| Teraspeed Modeling Services.
| http://www.teraspeed.com
[IBIS Ver]  3.2
[File Name] adc12d1600qml.ibs
[File Rev]  3.1
[Source]  Created by Teraspeed Consulting Group LLC
[Date]   05/03/2013
[Notes]   Quality Check of this IBIS model: Model Passes IBIS Check
   Model parses into ICX IS. Simulation done with Hyperlynx.
   1. MIN TYP MAX information is based on Temperature and
   Voltage characteristics only.
   2. Package data gained using TDA Systems IConnect Software.
[Disclaimer]
|[Disclaimer]
|(C) Copyright Texas Instruments Corporation 2013
|   All rights reserved
|   Texas Instruments Corporation hereby grants
|the user of this IBIS model a non-exclusive, nontransferable
|license to use this IBIS model under the following terms.
|Before using this IBIS model, the user should read this
|license.  If the user does not accept these terms,  the
|IBIS model should be returned to Texas Instruments within 30
|days.
|   The user is granted this license only to use the
|IBIS model and is not granted rights to sell, load, rent,
|lease or license the IBIS model in whole or in part, or in
|modified form to anyone other than user. User may modify
|the IBIS model to suit its specific applications but rights
|to derivative works and such modifications shall belong to
|Texas Instruments.
|   This IBIS model is provided on an "AS IS" basis and
|Texas Instruments makes absolutely no warranty with respect to
|the information contained herein.Texas Instruments DISCLAIMS AND
|CUSTOMER WAIVES ALL WARRANTIES, EXPRESS OR IMPLIED, INCLUDING
|WARRANTIES OF MERCHANTABILITY OR FITNESS FOR A PARTICULAR
|PURPOSE. The entire risk as to quality and performance is
|with the Customer. ACCORDINGLY, IN NO EVENT SHALL THE
|COMPANY BE LIABLE FOR ANY DAMAGES, WHETHER IN CONTRACT OR
|TORT,INCLUDING ANY LOST PROFITS OR OTHER INCIDENTAL,
|CONSEQUENTIAL, EXEMPLARY, OR PUNITIVE DAMAGES ARISING OUT
|OF THE USE OR APPLICATION OF THE IBIS model provided in
|this package.Further, Texas Instruments reserves the right to
|make changes without notice to any product herein to improve
|reliability, function, or design. Texas Instruments does not
|convey any license under patent rights or any other intellectual
|property rights, including those of third parties.
|   Texas Instruments is not obligated to provide maintenance
|or support for the licensed IBIS model.
| Use: Teraspeed Consulting Group LLC ("Teraspeed") has
| licensed IBIS models to specific integrated circuit
| suppliers ("IC Vendors") for use and distribution as
| follows: Each IC Vendor may use IBIS Models, and distribute
| them to IC Vendor's custumers to use solely for developing
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[Copyright]
| This file is the legal property of Texas Instruments and
| Teraspeed Copyright(c) 2013.
| All other rights are reserved.
[Component]   ADC12D1600QML
[Manufacturer] Texas Instruments
[Package]
| variable   typ   min   max
R_pkg  7.571E-03  2.653E-03   1.171E-02
L_pkg  3.048E-09  8.840E-10   1.031E-08
C_pkg  1.181E-12  2.940E-13   4.159E-12
[Pin] signal_name  model_name  R_pin  L_pin C_pin
A1   GND   GND   1.171E-02 8.840E-10 2.940E-13
A2   V_A   POWER   1.083E-02 8.840E-10 2.940E-13
A3   SDO   out_tri   1.000E-02 8.934E-09 3.594E-12
A4   TPM   input   9.232E-03 8.316E-09 3.340E-12
A5   NDM   input   8.534E-03 7.754E-09 3.110E-12
A6   V_A   POWER   7.917E-03 8.840E-10 2.940E-13
A7   GND   GND   7.392E-03 8.840E-10 2.940E-13
A8   V_E   POWER   6.969E-03 8.840E-10 2.940E-13
A9   GND_E   GND   6.659E-03 8.840E-10 2.940E-13
A10   DId0+   lvds_hs   6.469E-03 6.092E-09 2.429E-12
A11   V_DR   POWER   6.469E-03 8.840E-10 2.940E-13
A12   DId3+   lvds_hs   6.659E-03 6.244E-09 2.491E-12
A13   GND_DR   GND   6.969E-03 8.840E-10 2.940E-13
A14   DId6+   lvds_hs   7.392E-03 6.835E-09 2.733E-12
A15   V_DR   POWER   7.917E-03 8.840E-10 2.940E-13
A16   DId9+   lvds_hs   8.534E-03 7.754E-09 3.110E-12
A17   GND_DR   GND   9.232E-03 8.840E-10 2.940E-13
A18   DId11+   lvds_hs   1.000E-02 8.934E-09 3.594E-12
A19   DId11-   lvds_hs   1.083E-02 9.602E-09 3.868E-12
A20   GND_DR   GND   1.171E-02 8.840E-10 2.940E-13
B1   Vbg   term   1.083E-02 9.602E-09 3.868E-12
B2   GND   GND   9.900E-03 8.840E-10 2.940E-13
B3   ECEb   in_pu   9.020E-03 8.145E-09 3.271E-12
B4   SDI   input   8.201E-03 7.486E-09 3.000E-12
B5   CalRun   output   7.451E-03 6.882E-09 2.753E-12
B6   V_A   POWER   6.784E-03 8.840E-10 2.940E-13
B7   GND   GND   6.212E-03 8.840E-10 2.940E-13
B8   GND_E   GND   5.748E-03 8.840E-10 2.940E-13
B9   V_E   POWER   5.405E-03 8.840E-10 2.940E-13
B10   DId0-   lvds_hs   5.195E-03 5.066E-09 2.008E-12
B11   DId2+   lvds_hs   5.195E-03 5.066E-09 2.008E-12
B12   DId3-   lvds_hs   5.405E-03 5.235E-09 2.078E-12
B13   DId5+   lvds_hs   5.748E-03 5.511E-09 2.191E-12
B14   DId6-   lvds_hs   6.212E-03 5.884E-09 2.344E-12
B15   DId8+   lvds_hs   6.784E-03 6.345E-09 2.533E-12
B16   DId9-   lvds_hs   7.451E-03 6.882E-09 2.753E-12
B17   DId10+   lvds_hs   8.201E-03 7.486E-09 3.000E-12
B18   DI0+   lvds_hs   9.020E-03 8.145E-09 3.271E-12
B19   DI1+   lvds_hs   9.900E-03 8.853E-09 3.561E-12
B20   DI1-   lvds_hs   1.083E-02 9.602E-09 3.868E-12
C1   Rtrim+   term   1.000E-02 8.934E-09 3.594E-12
C2   GND   GND   9.020E-03 8.145E-09 3.271E-12
C3   Rext+   term   8.088E-03 7.395E-09 2.963E-12
C4   SCSb   input   7.212E-03 6.690E-09 2.674E-12
C5   SCLK   input   6.405E-03 6.040E-09 2.408E-12
C6   GND   GND   5.680E-03 8.840E-10 2.940E-13
C7   V_A   POWER   5.053E-03 8.840E-10 2.940E-13
C8   V_E   POWER   4.540E-03 8.840E-10 2.940E-13
C9   GND_E   GND   4.158E-03 8.840E-10 2.940E-13
C10   DId1+   lvds_hs   3.923E-03 4.042E-09 1.589E-12
C11   DId2-   lvds_hs   3.923E-03 4.042E-09 1.589E-12
C12   DId4+   lvds_hs   4.158E-03 4.232E-09 1.666E-12
C13   DId5-   lvds_hs   4.540E-03 4.539E-09 1.792E-12
C14   DId7+   lvds_hs   5.053E-03 4.951E-09 1.961E-12
C15   DId8-   lvds_hs   5.680E-03 5.456E-09 2.168E-12
C16   DId10-   lvds_hs   6.405E-03 6.040E-09 2.408E-12
C17   DI0-   lvds_hs   7.212E-03 6.690E-09 2.674E-12
C18   V_DR   POWER   8.088E-03 8.840E-10 2.940E-13
C19   DI12+   lvds_hs   9.020E-03 8.145E-09 3.271E-12
C20   DI12-   lvds_hs   1.000E-02 8.934E-09 3.594E-12
D1   V_A   POWER   9.232E-03 8.316E-09 3.340E-12
D2   Rtrim-   term   8.201E-03 7.486E-09 3.000E-12
D3   Rext-   term   7.212E-03 6.690E-09 2.674E-12
D4   GND   GND   6.276E-03 8.840E-10 2.940E-13
D5   GND   GND   5.405E-03 8.840E-10 2.940E-13
D6   CAL   input   4.615E-03 4.599E-09 1.817E-12
D7   Vbiasl   term   3.923E-03 4.042E-09 1.589E-12
D8   V_A   POWER   3.351E-03 8.840E-10 2.940E-13
D9   V_A   POWER   2.921E-03 8.840E-10 2.940E-13
D10   DId1-   lvds_hs   2.653E-03 3.020E-09 1.170E-12
D11   V_DR   POWER   2.653E-03 8.840E-10 2.940E-13
D12   DId4-   lvds_hs   2.921E-03 3.235E-09 1.258E-12
D13   GND_DR   GND   3.351E-03 8.840E-10 2.940E-13
D14   DId7-   lvds_hs   3.923E-03 4.042E-09 1.589E-12
D15   V_DR   POWER   4.615E-03 8.840E-10 2.940E-13
D16   GND_DR   GND   5.405E-03 8.840E-10 2.940E-13
D17   V_DR   POWER   6.276E-03 8.840E-10 2.940E-13
D18   DI3+   lvds_hs   7.212E-03 6.690E-09 2.674E-12
D19   DI4+   lvds_hs   8.201E-03 7.486E-09 3.000E-12
D20   DI4-   lvds_hs   9.232E-03 8.316E-09 3.340E-12
E1   V_A   POWER   8.534E-03 8.840E-10 2.940E-13
E2   Tdiode+   term   7.451E-03 6.882E-09 2.753E-12
E3   RSV1   NC   6.405E-03 6.040E-09 2.408E-12
E4   GND   GND   5.405E-03 8.840E-10 2.940E-13
E17   GND_DR   GND   5.405E-03 8.840E-10 2.940E-13
E18   DI3-   lvds_hs   6.405E-03 6.040E-09 2.408E-12
E19   DI5+   lvds_hs   7.451E-03 6.882E-09 2.753E-12
E20   DI5-   lvds_hs   8.534E-03 7.754E-09 3.110E-12
F1   V_A   POWER   7.917E-03 8.840E-10 2.940E-13
F2   GND_TC   GND   6.784E-03 8.840E-10 2.940E-13
F3   Tdiode-   term   5.680E-03 5.456E-09 2.168E-12
F4   RSV2   NC   4.615E-03 4.599E-09 1.817E-12
F17   GND_DR   GND   4.615E-03 8.840E-10 2.940E-13
F18   DI6+   lvds_hs   5.680E-03 5.456E-09 2.168E-12
F19   DI6-   lvds_hs   6.784E-03 6.345E-09 2.533E-12
F20   GND_DR   GND   7.917E-03 8.840E-10 2.940E-13
G1   V_TC   POWER   7.392E-03 8.840E-10 2.940E-13
G2   GND_TC   GND   6.212E-03 8.840E-10 2.940E-13
G3   V_TC   POWER   5.053E-03 8.840E-10 2.940E-13
G4   V_TC   POWER   3.923E-03 8.840E-10 2.940E-13
G17   DI7+   lvds_hs   3.923E-03 8.840E-10 2.940E-13
G18   DI7-   lvds_hs   5.053E-03 8.951E-10 2.961E-13
G19   DI8+   lvds_hs   6.212E-03 5.884E-09 2.344E-12
G20   DI8-   lvds_hs   7.392E-03 6.835E-09 2.733E-12
H1   Vinl+   term   6.969E-03 6.494E-09 2.594E-12
H2   V_TC   POWER   5.748E-03 8.840E-10 2.940E-13
H3   GND_TC   GND   4.540E-03 8.840E-10 2.940E-13
H4   V_A   POWER   3.351E-03 8.840E-10 2.940E-13
H17   DI9+   lvds_hs   3.351E-03 3.581E-09 1.400E-12
H18   DI9-   lvds_hs   4.540E-03 4.539E-09 1.792E-12
H19   DI10+   lvds_hs   5.748E-03 5.511E-09 2.191E-12
H20   DI10-   lvds_hs   6.969E-03 6.494E-09 2.594E-12
J1   Vinl-   term   6.659E-03 6.244E-09 2.491E-12
J2   GND_TC   GND   5.405E-03 8.840E-10 2.940E-13
J3   V_TC   POWER   4.158E-03 8.840E-10 2.940E-13
J4   VbiasI   term   2.921E-03 3.235E-09 1.258E-12
J17   V_DR   POWER   2.921E-03 8.840E-10 2.940E-13
J18   DI11+   lvds_hs   4.158E-03 4.232E-09 1.666E-12
J19   DI11-   lvds_hs   5.405E-03 5.235E-09 2.078E-12
J20   V_DR   POWER   6.659E-03 8.840E-10 2.940E-13
K1   GND   GND   6.469E-03 8.840E-10 2.940E-13
K2   VbiasI   term   5.195E-03 5.066E-09 2.008E-12
K3   V_TC   POWER   3.923E-03 8.840E-10 2.940E-13
K4   GND_TC   GND   2.653E-03 8.840E-10 2.940E-13
K17   ORI+   lvds_hs   2.653E-03 3.020E-09 1.170E-12
K18   ORI-   lvds_hs   3.923E-03 4.042E-09 1.589E-12
K19   DCLKI+   lvds_hs   5.195E-03 5.066E-09 2.008E-12
K20   DCLKI-   lvds_hs   6.469E-03 6.092E-09 2.429E-12
L1   GND   GND   6.469E-03 8.840E-10 2.940E-13
L2   VbiasQ   term   5.195E-03 5.066E-09 2.008E-12
L3   V_TC   POWER   3.923E-03 8.840E-10 2.940E-13
L4   GND_TC   GND   2.653E-03 8.840E-10 2.940E-13
L17   ORQ+   lvds_hs   2.653E-03 3.020E-09 1.170E-12
L18   ORQ-   lvds_hs   3.923E-03 4.042E-09 1.589E-12
L19   DCLKQ+   lvds_hs   5.195E-03 5.066E-09 2.008E-12
L20   DCLKQ-   lvds_hs   6.469E-03 6.092E-09 2.429E-12
M1   VinQ-   term   6.659E-03 6.244E-09 2.491E-12
M2   GND_TC   GND   5.405E-03 8.840E-10 2.940E-13
M3   V_TC   POWER   4.158E-03 8.840E-10 2.940E-13
M4   VbiasQ   term   2.921E-03 3.235E-09 1.258E-12
M17   GND_DR   GND   2.921E-03 8.840E-10 2.940E-13
M18   DQ11+   lvds_hs   4.158E-03 4.232E-09 1.666E-12
M19   DQ11-   lvds_hs   5.405E-03 5.235E-09 2.078E-12
M20   GND_DR   GND   6.659E-03 8.840E-10 2.940E-13
N1   VinQ+   term   6.969E-03 6.494E-09 2.594E-12
N2   V_TC   POWER   5.748E-03 8.840E-10 2.940E-13
N3   GND_TC   GND   4.540E-03 8.840E-10 2.940E-13
N4   V_A   POWER   3.351E-03 8.840E-10 2.940E-13
N17   DQ9+   lvds_hs   3.351E-03 3.581E-09 1.400E-12
N18   DQ9-   lvds_hs   4.540E-03 4.539E-09 1.792E-12
N19   DQ10+   lvds_hs   5.748E-03 5.511E-09 2.191E-12
N20   DQ10-   lvds_hs   6.969E-03 6.494E-09 2.594E-12
P1   V_TC   POWER   7.392E-03 8.840E-10 2.940E-13
P2   GND_TC   GND   6.212E-03 8.840E-10 2.940E-13
P3   V_TC   POWER   5.053E-03 8.840E-10 2.940E-13
P4   V_TC   POWER   3.923E-03 8.840E-10 2.940E-13
P17   DQ7+   lvds_hs   3.923E-03 4.042E-09 1.589E-12
P18   DQ7-   lvds_hs   5.053E-03 4.951E-09 1.961E-12
P19   DQ8+   lvds_hs   6.212E-03 5.884E-09 2.344E-12
P20   DQ8-   lvds_hs   7.392E-03 6.835E-09 2.733E-12
R1   V_A   POWER   7.917E-03 8.840E-10 2.940E-13
R2   GND_TC   GND   6.784E-03 8.840E-10 2.940E-13
R3   V_TC   POWER   5.680E-03 8.840E-10 2.940E-13
R4   V_TC   POWER   4.615E-03 8.840E-10 2.940E-13
R17   V_DR   POWER   4.615E-03 8.840E-10 2.940E-13
R18   DQ6+   lvds_hs   5.680E-03 5.456E-09 2.168E-12
R19   DQ6-   lvds_hs   6.784E-03 6.345E-09 2.533E-12
R20   V_DR   POWER   7.917E-03 8.840E-10 2.940E-13
T1   V_A   POWER   8.534E-03 8.840E-10 2.940E-13
T2   GND_TC   GND   7.451E-03 8.840E-10 2.940E-13
T3   GND_TC   GND   6.405E-03 8.840E-10 2.940E-13
T4   GND   GND   5.405E-03 8.840E-10 2.940E-13
T17   V_DR   POWER   5.405E-03 8.840E-10 2.940E-13
T18   DQ3-   lvds_hs   6.405E-03 6.040E-09 2.408E-12
T19   DQ5+   lvds_hs   7.451E-03 6.882E-09 2.753E-12
T20   DQ5-   lvds_hs   8.534E-03 7.754E-09 3.110E-12
U1   GND_TC   GND   9.232E-03 8.840E-10 2.940E-13
U2   CLK+   in_clk   8.201E-03 7.486E-09 3.000E-12
U3   PDI   in_pu   7.212E-03 6.690E-09 2.674E-12
U4   GND   GND   6.276E-03 8.840E-10 2.940E-13
U5   GND   GND   5.405E-03 8.840E-10 2.940E-13
U6   RCOut1-   lvds_ls   4.615E-03 4.599E-09 1.817E-12
U7   VbiasQ   term   3.923E-03 4.042E-09 1.589E-12
U8   V_A   POWER   3.351E-03 8.840E-10 2.940E-13
U9   V_A   POWER   2.921E-03 8.840E-10 2.940E-13
U10   DQd1-   lvds_hs   2.653E-03 3.020E-09 1.170E-12
U11   V_DR   POWER   2.653E-03 8.840E-10 2.940E-13
U12   DQd4-   lvds_hs   2.921E-03 3.235E-09 1.258E-12
U13   GND_DR   GND   3.351E-03 8.840E-10 2.940E-13
U14   DQd7-   lvds_hs   3.923E-03 4.042E-09 1.589E-12
U15   V_DR   POWER   4.615E-03 8.840E-10 2.940E-13
U16   V_DR   POWER   5.405E-03 8.840E-10 2.940E-13
U17   GND_DR   GND   6.276E-03 8.840E-10 2.940E-13
U18   DQ3+   lvds_hs   7.212E-03 6.690E-09 2.674E-12
U19   DQ4+   lvds_hs   8.201E-03 7.486E-09 3.000E-12
U20   DQ4-   lvds_hs   9.232E-03 8.316E-09 3.340E-12
V1   CLK-   in_clk   1.000E-02 8.934E-09 3.594E-12
V2   DCLK_RST+ in_clk   9.020E-03 8.145E-09 3.271E-12
V3   PDQ   in_pu   8.088E-03 7.395E-09 2.963E-12
V4   LSPSM   input   7.212E-03 6.690E-09 2.674E-12
V5   DES   input   6.405E-03 6.040E-09 2.408E-12
V6   RCOut2+   lvds_ls   5.680E-03 5.456E-09 2.168E-12
V7   RCOut2-   lvds_ls   5.053E-03 4.951E-09 1.961E-12
V8   V_E   POWER   4.540E-03 8.840E-10 2.940E-13
V9   GND_E   GND   4.158E-03 8.840E-10 2.940E-13
V10   DQd1+   lvds_hs   3.923E-03 4.042E-09 1.589E-12
V11   DQd02-   lvds_hs   3.923E-03 4.042E-09 1.589E-12
V12   DQd4+   lvds_hs   4.158E-03 4.232E-09 1.666E-12
V13   DQd5-   lvds_hs   4.540E-03 4.539E-09 1.792E-12
V14   DQd7+   lvds_hs   5.053E-03 4.951E-09 1.961E-12
V15   DQd8-   lvds_hs   5.680E-03 5.456E-09 2.168E-12
V16   DQd10-   lvds_hs   6.405E-03 6.040E-09 2.408E-12
V17   DQ0-   lvds_hs   7.212E-03 6.690E-09 2.674E-12
V18   GND_DR   GND   8.088E-03 8.840E-10 2.940E-13
V19   DQ2+   lvds_hs   9.020E-03 8.145E-09 3.271E-12
V20   DQ2-   lvds_hs   1.000E-02 8.934E-09 3.594E-12
W1   DCLK_RST- in_clk   1.083E-02 9.602E-09 3.868E-12
W2   GND   GND   9.900E-03 8.840E-10 2.940E-13
W3   RSV   NC   9.020E-03 8.145E-09 3.271E-12
W4   DDRPh   input   8.201E-03 7.486E-09 3.000E-12
W5   RCLK-   in_clk   7.451E-03 6.882E-09 2.753E-12
W6   V_A   POWER   6.784E-03 8.840E-10 2.940E-13
W7   GND   GND   6.212E-03 8.840E-10 2.940E-13
W8   GND_E   GND   5.748E-03 8.840E-10 2.940E-13
W9   V_E   POWER   5.405E-03 8.840E-10 2.940E-13
W10   DQd0-   lvds_hs   5.195E-03 5.066E-09 2.008E-12
W11   DQd2+   lvds_hs   5.195E-03 5.066E-09 2.008E-12
W12   DQd3-   lvds_hs   5.405E-03 5.235E-09 2.078E-12
W13   DQd5+   lvds_hs   5.748E-03 5.511E-09 2.191E-12
W14   DQd6-   lvds_hs   6.212E-03 5.884E-09 2.344E-12
W15   DQd8+   lvds_hs   6.784E-03 6.345E-09 2.533E-12
W16   DQd9-   lvds_hs   7.451E-03 6.882E-09 2.753E-12
W17   DQd10+   lvds_hs   8.201E-03 7.486E-09 3.000E-12
W18   DQ0+   lvds_hs   9.020E-03 8.145E-09 3.271E-12
W19   DQ1+   lvds_hs   9.900E-03 8.853E-09 3.561E-12
W20   DQ1-   lvds_hs   1.083E-02 9.602E-09 3.868E-12
Y1   GND   GND   1.171E-02 8.840E-10 2.940E-13
Y2   V_A   POWER   1.083E-02 8.840E-10 2.940E-13
Y3   FSR   input   1.000E-02 8.934E-09 3.594E-12
Y4   RCLK+   in_clk   9.232E-03 8.316E-09 3.340E-12
Y5   RCOut1+   lvds_ls   8.534E-03 7.754E-09 3.110E-12
Y6   V_A   POWER   7.917E-03 8.840E-10 2.940E-13
Y7   GND   GND   7.392E-03 8.840E-10 2.940E-13
Y8   V_E   POWER   6.969E-03 8.840E-10 2.940E-13
Y9   GND_E   GND   6.659E-03 8.840E-10 2.940E-13
Y10   DQd0+   lvds_hs   6.469E-03 6.092E-09 2.429E-12
Y11   V_DR   POWER   6.469E-03 8.840E-10 2.940E-13
Y12   DQd3+   lvds_hs   6.659E-03 6.244E-09 2.491E-12
Y13   GND_DR   GND   6.969E-03 8.840E-10 2.940E-13
Y14   DQd6+   lvds_hs   7.392E-03 6.835E-09 2.733E-12
Y15   V_DR   POWER   7.917E-03 8.840E-10 2.940E-13
Y16   DQd9+   lvds_hs   8.534E-03 7.754E-09 3.110E-12
Y17   GND_DR   GND   9.232E-03 8.840E-10 2.940E-13
Y18   DQd11+   lvds_hs   1.000E-02 8.934E-09 3.594E-12
Y19   DQd11-   lvds_hs   1.083E-02 9.602E-09 3.868E-12
Y20   GND_DR   GND   1.171E-02 1.031E-08 4.159E-12
AA2   GND   GND   1.000E-02 8.840E-10 2.940E-13
AA3   GND   GND   1.000E-02 8.840E-10 2.940E-13
AA4   GND   GND   1.000E-02 8.840E-10 2.940E-13
AA5   GND   GND   1.000E-02 8.840E-10 2.940E-13
AA6   GND   GND   1.000E-02 8.840E-10 2.940E-13
AA7   GND   GND   1.000E-02 8.840E-10 2.940E-13
AA8   GND   GND   1.000E-02 8.840E-10 2.940E-13
AA9   GND   GND   1.000E-02 8.840E-10 2.940E-13
AA10  GND   GND   1.000E-02 8.840E-10 2.940E-13
AA11  GND   GND   1.000E-02 8.840E-10 2.940E-13
AB1   GND   GND   1.000E-02 8.840E-10 2.940E-13
AB2   GND   GND   1.000E-02 8.840E-10 2.940E-13
AB3   GND   GND   1.000E-02 8.840E-10 2.940E-13
AB4   GND   GND   1.000E-02 8.840E-10 2.940E-13
AB5   GND   GND   1.000E-02 8.840E-10 2.940E-13
AB6   GND   GND   1.000E-02 8.840E-10 2.940E-13
AB7   GND   GND   1.000E-02 8.840E-10 2.940E-13
AB8   GND   GND   1.000E-02 8.840E-10 2.940E-13
AB9   GND   GND   1.000E-02 8.840E-10 2.940E-13
AB10  GND   GND   1.000E-02 8.840E-10 2.940E-13
AB11  GND   GND   1.000E-02 8.840E-10 2.940E-13
AC1   GND   GND   1.000E-02 8.840E-10 2.940E-13
AC2   GND   GND   1.000E-02 8.840E-10 2.940E-13
AC3   GND   GND   1.000E-02 8.840E-10 2.940E-13
AC4   GND   GND   1.000E-02 8.840E-10 2.940E-13
AC5   GND   GND   1.000E-02 8.840E-10 2.940E-13
AC6   GND   GND   1.000E-02 8.840E-10 2.940E-13
AC7   GND   GND   1.000E-02 8.840E-10 2.940E-13
AC8   GND   GND   1.000E-02 8.840E-10 2.940E-13
AC9   GND   GND   1.000E-02 8.840E-10 2.940E-13
AC10  GND   GND   1.000E-02 8.840E-10 2.940E-13
AC11  GND   GND   1.000E-02 8.840E-10 2.940E-13
AD1   GND   GND   1.000E-02 8.840E-10 2.940E-13
AD2   GND   GND   1.000E-02 8.840E-10 2.940E-13
AD3   GND   GND   1.000E-02 8.840E-10 2.940E-13
AD4   GND   GND   1.000E-02 8.840E-10 2.940E-13
AD5   GND   GND   1.000E-02 8.840E-10 2.940E-13
AD6   GND   GND   1.000E-02 8.840E-10 2.940E-13
AD7   GND   GND   1.000E-02 8.840E-10 2.940E-13
AD8   GND   GND   1.000E-02 8.840E-10 2.940E-13
AD9   GND   GND   1.000E-02 8.840E-10 2.940E-13
AD10  GND   GND   1.000E-02 8.840E-10 2.940E-13
AD11  GND   GND   1.000E-02 8.840E-10 2.940E-13
AE1   GND   GND   1.000E-02 8.840E-10 2.940E-13
AE2   GND   GND   1.000E-02 8.840E-10 2.940E-13
AE3   GND   GND   1.000E-02 8.840E-10 2.940E-13
AE4   GND   GND   1.000E-02 8.840E-10 2.940E-13
AE5   GND   GND   1.000E-02 8.840E-10 2.940E-13
AE6   GND   GND   1.000E-02 8.840E-10 2.940E-13
AE7   GND   GND   1.000E-02 8.840E-10 2.940E-13
AE8   GND   GND   1.000E-02 8.840E-10 2.940E-13
AE9   GND   GND   1.000E-02 8.840E-10 2.940E-13
AE10  GND   GND   1.000E-02 8.840E-10 2.940E-13
AE11  GND   GND   1.000E-02 8.840E-10 2.940E-13
AF1   GND   GND   1.000E-02 8.840E-10 2.940E-13
AF2   GND   GND   1.000E-02 8.840E-10 2.940E-13
AF3   GND   GND   1.000E-02 8.840E-10 2.940E-13
AF4   GND   GND   1.000E-02 8.840E-10 2.940E-13
AF5   GND   GND   1.000E-02 8.840E-10 2.940E-13
AF6   GND   GND   1.000E-02 8.840E-10 2.940E-13
AF7   GND   GND   1.000E-02 8.840E-10 2.940E-13
AF8   GND   GND   1.000E-02 8.840E-10 2.940E-13
AF9   GND   GND   1.000E-02 8.840E-10 2.940E-13
AF10  GND   GND   1.000E-02 8.840E-10 2.940E-13
AF11  GND   GND   1.000E-02 8.840E-10 2.940E-13
AG1   GND   GND   1.000E-02 8.840E-10 2.940E-13
AG2   GND   GND   1.000E-02 8.840E-10 2.940E-13
AG3   GND   GND   1.000E-02 8.840E-10 2.940E-13
AG4   GND   GND   1.000E-02 8.840E-10 2.940E-13
AG5   GND   GND   1.000E-02 8.840E-10 2.940E-13
AG6   GND   GND   1.000E-02 8.840E-10 2.940E-13
AG7   GND   GND   1.000E-02 8.840E-10 2.940E-13
AG8   GND   GND   1.000E-02 8.840E-10 2.940E-13
AG9   GND   GND   1.000E-02 8.840E-10 2.940E-13
AG10  GND   GND   1.000E-02 8.840E-10 2.940E-13
AG11  GND   GND   1.000E-02 8.840E-10 2.940E-13
AH1   GND   GND   1.000E-02 8.840E-10 2.940E-13
AH2   GND   GND   1.000E-02 8.840E-10 2.940E-13
AH3   GND   GND   1.000E-02 8.840E-10 2.940E-13
AH4   GND   GND   1.000E-02 8.840E-10 2.940E-13
AH5   GND   GND   1.000E-02 8.840E-10 2.940E-13
AH6   GND   GND   1.000E-02 8.840E-10 2.940E-13
AH7   GND   GND   1.000E-02 8.840E-10 2.940E-13
AH8   GND   GND   1.000E-02 8.840E-10 2.940E-13
AH9   GND   GND   1.000E-02 8.840E-10 2.940E-13
AH10  GND   GND   1.000E-02 8.840E-10 2.940E-13
AH11  GND   GND   1.000E-02 8.840E-10 2.940E-13
AJ1   GND   GND   1.000E-02 8.840E-10 2.940E-13
AJ2   GND   GND   1.000E-02 8.840E-10 2.940E-13
AJ3   GND   GND   1.000E-02 8.840E-10 2.940E-13
AJ4   GND   GND   1.000E-02 8.840E-10 2.940E-13
AJ5   GND   GND   1.000E-02 8.840E-10 2.940E-13
AJ6   GND   GND   1.000E-02 8.840E-10 2.940E-13
AJ7   GND   GND   1.000E-02 8.840E-10 2.940E-13
AJ8   GND   GND   1.000E-02 8.840E-10 2.940E-13
AJ9   GND   GND   1.000E-02 8.840E-10 2.940E-13
AJ10  GND   GND   1.000E-02 8.840E-10 2.940E-13
AJ11  GND   GND   1.000E-02 8.840E-10 2.940E-13
AK1   GND   GND   1.000E-02 8.840E-10 2.940E-13
AK2   GND   GND   1.000E-02 8.840E-10 2.940E-13
AK3   GND   GND   1.000E-02 8.840E-10 2.940E-13
AK4   GND   GND   1.000E-02 8.840E-10 2.940E-13
AK5   GND   GND   1.000E-02 8.840E-10 2.940E-13
AK6   GND   GND   1.000E-02 8.840E-10 2.940E-13
AK7   GND   GND   1.000E-02 8.840E-10 2.940E-13
AK8   GND   GND   1.000E-02 8.840E-10 2.940E-13
AK9   GND   GND   1.000E-02 8.840E-10 2.940E-13
AK10  GND   GND   1.000E-02 8.840E-10 2.940E-13
AK11  GND   GND   1.000E-02 8.840E-10 2.940E-13
AL1   GND   GND   1.000E-02 8.840E-10 2.940E-13
AL2   GND   GND   1.000E-02 8.840E-10 2.940E-13
AL3   GND   GND   1.000E-02 8.840E-10 2.940E-13
AL4   GND   GND   1.000E-02 8.840E-10 2.940E-13
AL5   GND   GND   1.000E-02 8.840E-10 2.940E-13
AL6   GND   GND   1.000E-02 8.840E-10 2.940E-13
AL7   GND   GND   1.000E-02 8.840E-10 2.940E-13
AL8   GND   GND   1.000E-02 8.840E-10 2.940E-13
AL9   GND   GND   1.000E-02 8.840E-10 2.940E-13
AL10  GND   GND   1.000E-02 8.840E-10 2.940E-13
AL11  GND   GND   1.000E-02 8.840E-10 2.940E-13
[Diff Pin] inv_pin vdiff tdelay_typ tdelay_min tdelay_max
U2   V1   200mV NA   NA   NA
V2   W1   200mV NA   NA   NA
Y4   W5   200mV NA   NA   NA
A10   B10   NA   NA   NA   NA
A12   B12   NA   NA   NA   NA
A14   B14   NA   NA   NA   NA
A16   B16   NA   NA   NA   NA
A18   A19   NA   NA   NA   NA
B11   C11   NA   NA   NA   NA
B13   C13   NA   NA   NA   NA
B15   C15   NA   NA   NA   NA
B17   C16   NA   NA   NA   NA
B18   C17   NA   NA   NA   NA
B19   B20   NA   NA   NA   NA
C1   D2   NA   NA   NA   NA
C10   D10   NA   NA   NA   NA
C12   D12   NA   NA   NA   NA
C14   D14   NA   NA   NA   NA
C19   C20   NA   NA   NA   NA
C3   D3   NA   NA   NA   NA
D18   E18   NA   NA   NA   NA
D19   D20   NA   NA   NA   NA
E19   E20   NA   NA   NA   NA
E2   F3   NA   NA   NA   NA
F18   F19   NA   NA   NA   NA
G17   G18   NA   NA   NA   NA
G19   G20   NA   NA   NA   NA
H1   J1   NA   NA   NA   NA
H17   H18   NA   NA   NA   NA
H19   H20   NA   NA   NA   NA
J18   J19   NA   NA   NA   NA
K17   K18   NA   NA   NA   NA
K19   K20   NA   NA   NA   NA
L17   L18   NA   NA   NA   NA
L19   L20   NA   NA   NA   NA
M18   M19   NA   NA   NA   NA
N1   M1   NA   NA   NA   NA
N17   N18   NA   NA   NA   NA
N19   N20   NA   NA   NA   NA
P17   P18   NA   NA   NA   NA
P19   P20   NA   NA   NA   NA
R18   R19   NA   NA   NA   NA
T19   T20   NA   NA   NA   NA
U18   T18   NA   NA   NA   NA
U19   U20   NA   NA   NA   NA
V10   U10   NA   NA   NA   NA
V12   U12   NA   NA   NA   NA
V14   U14   NA   NA   NA   NA
V19   V20   NA   NA   NA   NA
V6   V7   NA   NA   NA   NA
W11   V11   NA   NA   NA   NA
W13   V13   NA   NA   NA   NA
W15   V15   NA   NA   NA   NA
W17   V16   NA   NA   NA   NA
W18   V17   NA   NA   NA   NA
W19   W20   NA   NA   NA   NA
Y10   W10   NA   NA   NA   NA
Y12   W12   NA   NA   NA   NA
Y14   W14   NA   NA   NA   NA
Y16   W16   NA   NA   NA   NA
Y18   Y19   NA   NA   NA   NA
Y5   U6   NA   NA   NA   NA
[Series Pin Mapping] pin_2 model_name function_table_group
H1   J1   100_ohm
N1   M1   100_ohm
U2   V1   100_ohm
V2   W1   100_ohm
Y4   W5   100_ohm
C3   D3   3300_ohm
C1   D2   3300_ohm
[Model Selector]  lvds_hs
lvds_lo_vbgf   output voltage=lo, vbg=floating
lvds_hi_vbgf   output voltage=hi, vbg=floating
lvds_lo_vbg1   output voltage=lo, vbg=hi
lvds_hi_vbg1   output voltage=hi, vbg=hi
[Model]   100_ohm
Model_type   Series
C_comp   0  0  0
[Temperature Range]   25   85   -40
|   typ   min   max
[Voltage Range]  1.9V 1.8V 2.0V
[R series]   100   94   106
[Model]   3300_ohm
Model_type   Series
C_comp   0  0  0
[Temperature Range]   25   85   -40
|   typ   min   max
[Voltage Range]  1.9V   1.8V   2.0V
[R series]   3300   3300   3300
[Model] term
Model_type Terminator
C_comp   0  0  0
| variable   typ   min   max
[Voltage Range]   1.900E+00   1.800E+00   2.000E+00
[POWER Clamp Reference]  1.900E+00   1.800E+00   2.000E+00
[GND Clamp Reference]   0.00000V   0.00000V   0.00000V
[Temperature Range]   25   85   -40
| Models and submodels in the file (13): in_clk (Input), in_pu (Input), input (Input), lvds_hi_vbg1 (Output), lvds_hi_vbgf (Output), lvds_lo_vbg1 (Output), lvds_lo_vbgf (Output), lvds_ls (Output), out_tri (3-state), output (Output), 100_ohm (Series), 3300_ohm (Series), term (Terminator)
